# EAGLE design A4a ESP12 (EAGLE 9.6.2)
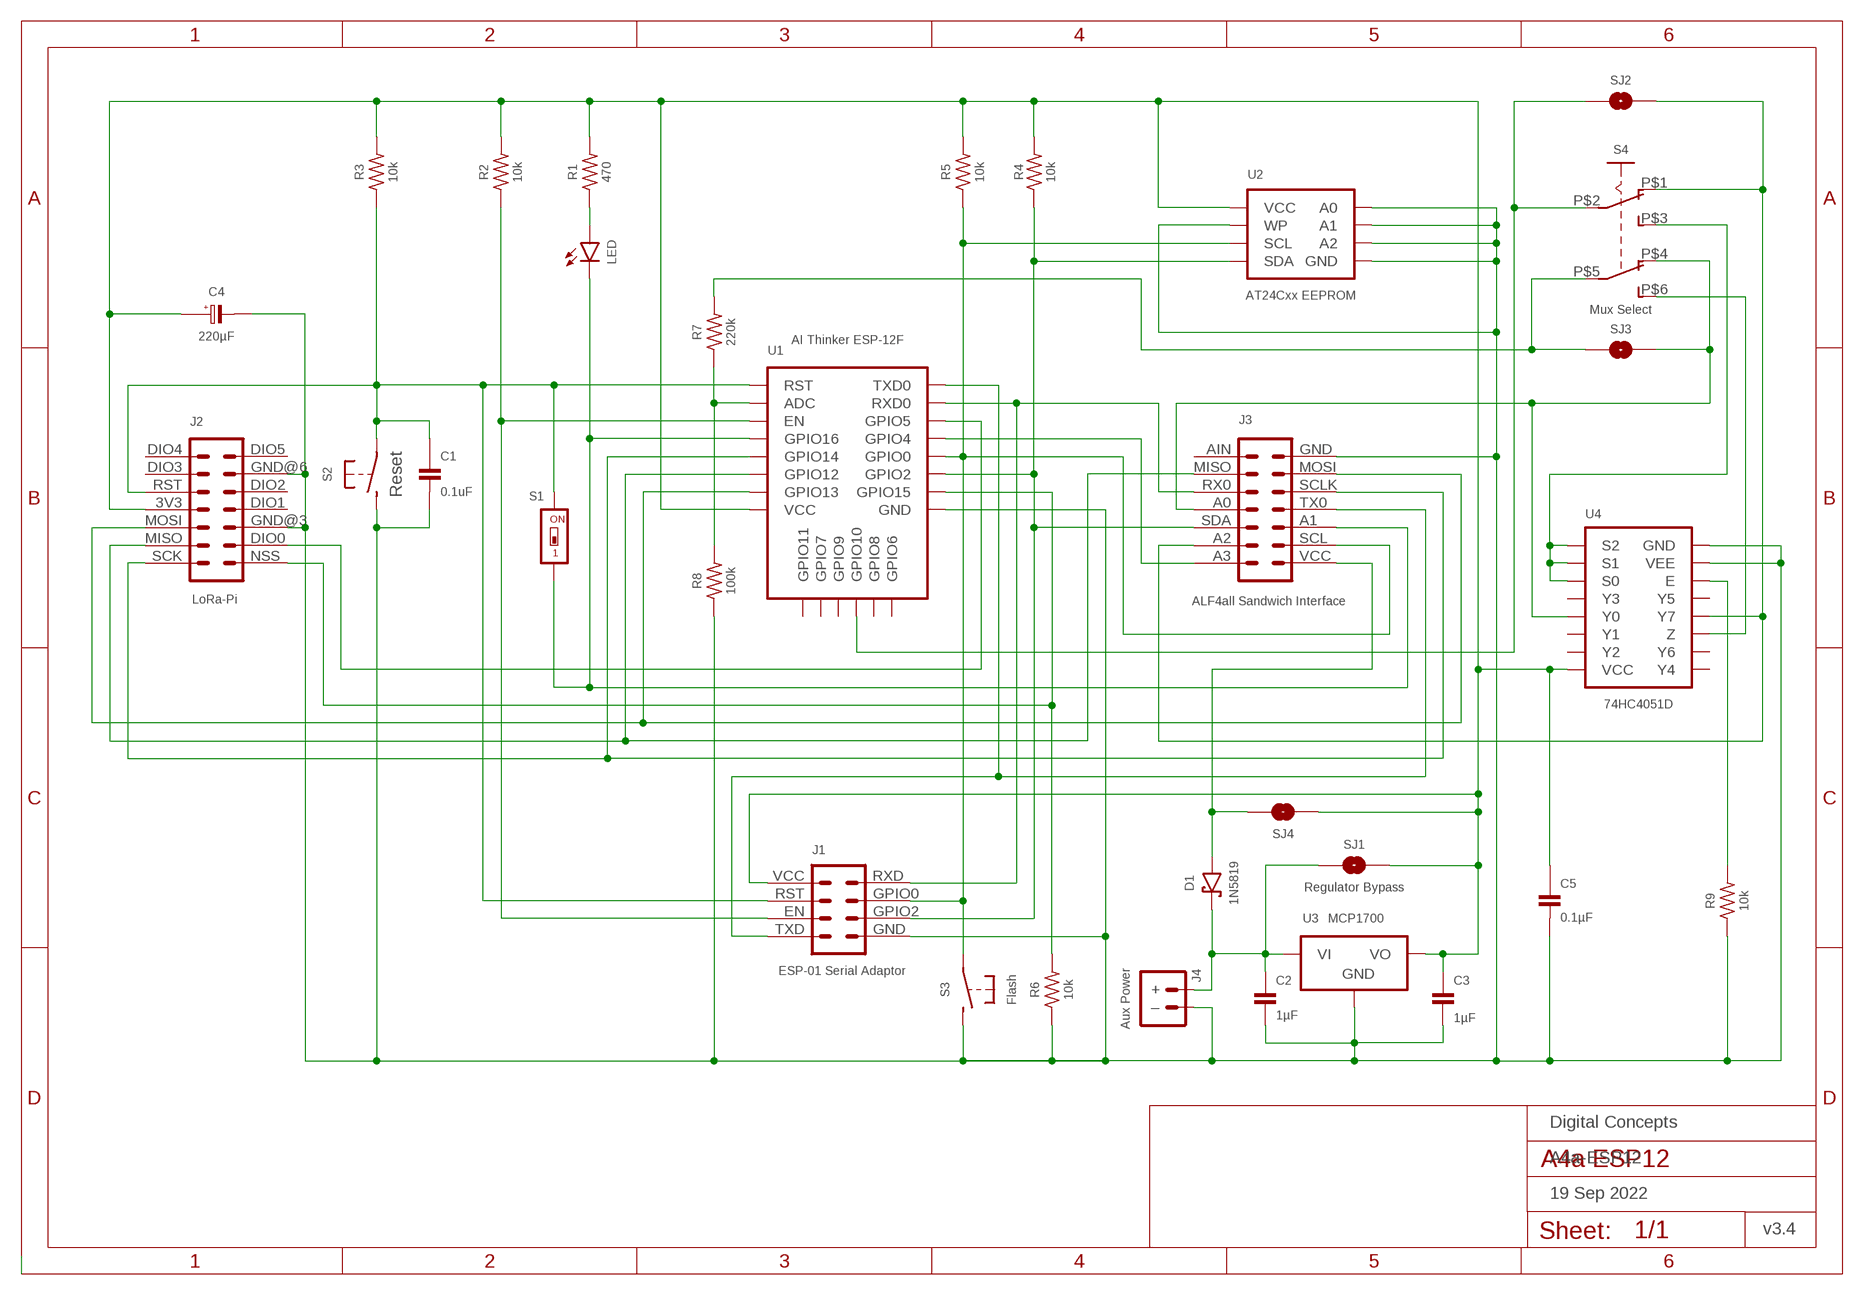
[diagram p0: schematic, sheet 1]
FRAME1 (A4L-LOC): DATE: 19 Sep 2022; OWNER: Digital Concepts; TITLE: A4a-ESP12; VERSION: v3.4

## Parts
C1  0.1uF  CAPACITOR-0805  [C0805]
C2  1µF  CAPACITOR  [C0805@1]
C3  1µF  CAPACITOR  [C0805@1]
C4  220µF  CAPACITOR-TANTALUM-3528  [C3528-21]
C5  0.1µF  CAPACITOR-0805  [C0805]
D1  1N5819  DIODE-SCHOTTKY-1N5819  [SOD-123]
J1  ESP-01 Serial Adaptor  ESP-01-SERIAL-ADAPTOR  [CONN_2X4-ESP-01-SERIAL]
J2  LoRa-Pi  RFM95W-PI-HEADER  [RFM95W-PI]
J3  ALF4all Sandwich Interface  HEADER-2X7-ALF4ALL-PROCESSOR-B  [CONN_2X7-ALF4ALL-PROCESSOR-B]
J4  Aux Power  JST-PH2.0-2-MALE-HORIZONTALJST-PTH-2  [JST-PH2.0-2-HORIZONTAL]
LED  LEDCHIP-LED0805  [CHIP-LED0805]
R1  470  RESISTORR0805  [R0805]
R2  10k  RESISTORR0805  [R0805]
R3  10k  RESISTORR0805  [R0805]
R4  10k  RESISTORR0805  [R0805]
R5  10k  RESISTORR0805  [R0805]
R6  10k  RESISTORR0805  [R0805]
R7  220k  RESISTORR0805  [R0805]
R8  100k  RESISTORR0805  [R0805]
R9  10k  RESISTORR0805  [R0805]
S1  Wake  SWITCH-DIP-SWS001  [SMD-001]
S2  Reset  SWITCH-MOMENTARY-2-PIN  [SWITCH-2-PAD]
S3  Flash  SWITCH-MOMENTARY-2-PIN  [SWITCH-2-PAD]
S4  Mux Select  SWITCH-SLIDE-DPDT  [SWITCH-DPDT-SMD]
SJ1  Regulator Bypass  SJ  [SJ]
SJ2  SJ  [SJ]
SJ3  SJ  [SJ]
SJ4  SJ  [SJ]
U1  AI Thinker ESP-12F  ESP-12E/F  [ESP-12E/F]
U2  AT24Cxx EEPROM  AT24CXX-EEPROM  [SOP-8]
U3  MCP1700  [SOT-23-3]
U4  74HC4051D  [SOP16]

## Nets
GND: C1.2 C2.2 C3.2 C4.2(-) C5.2 J1.GND J2.GND@3 J2.GND@6 J3.GND J4.-(–) R6.1 R8.1 R9.1 S2.P$2(S) S3.P$2(S) U1.GND U2.P$1(A0) U2.P$2(A1) U2.P$3(A2) U2.P$4(GND) U2.P$7(WP) U3.1(GND) U4.7(VEE) U4.8(GND)
N$1: S4.P$2(P1) SJ2.1 U1.GPIO10
N$2: J2.NSS R6.2 U1.GPIO15
N$3: J2.SCK J3.SCLK U1.GPIO14
N$4: C1.1 J1.RST J2.RST R3.1 S1.2 S2.P$1(P) U1.RST
N$5: J2.MISO J3.MISO U1.GPIO12
N$6: J2.MOSI J3.MOSI U1.GPIO13
N$7: R7.1 R8.2 U1.ADC
N$8: J1.EN R2.1 U1.EN
N$9: D1.A J3.VCC SJ4.1
N$10: J1.TXD J3.TX0 U1.TXD0
N$11: J1.GPIO2 J3.SDA R4.1 U1.GPIO2 U2.P$5(SDA)
N$12: J3.A3 U1.GPIO4
N$13: J1.GPIO0 J3.SCL R5.1 S3.P$1(P) U1.GPIO0 U2.P$6(SCL)
N$14: LED.A R1.1
N$15: J3.A1 LED.C S1.1 U1.GPIO16
N$16: J1.RXD J3.RX0 U1.RXD0
N$17: R9.2 U4.6(E)
N$19: J2.DIO0 U1.GPIO5
N$20: J3.A2 S4.P$1(O1) SJ2.2 U4.4(Y7)
N$21: J3.A0 S4.P$4(O2) SJ3.2 U4.13(Y0)
N$22: S4.P$6(S2) U4.3(Z)
N$23: S4.P$3(S1) U4.9(S2) U4.10(S1) U4.11(S0)
N$25: R7.2 S4.P$5(P2) SJ3.1
N$26: C2.1 D1.C J4.+ SJ1.1 U3.3(VI)
VCC: C3.1 C4.1(+) C5.1 J1.VCC J2.3V3 R1.2 R2.2 R3.2 R4.2 R5.2 SJ1.2 SJ4.2 U1.VCC U2.P$8(VCC) U3.2(VO) U4.16(VCC)
Unconnected: J2.DIO1 J2.DIO2 J2.DIO3 J2.DIO4 J2.DIO5 J3.AIN U1.CS0(GPIO11) U1.GPIO9 U1.MISO(GPIO7) U1.MOSI(GPIO8) U1.SCLK(GPIO6) U4.1(Y4) U4.2(Y6) U4.5(Y5) U4.12(Y3) U4.14(Y1) U4.15(Y2)

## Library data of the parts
C1 C5 = digitalconcepts:CAPACITOR-0805: 0805 Capacitor
C2 C3 = digitalconcepts:CAPACITOR: 0805 Capacitor
C4 = digitalconcepts:CAPACITOR-TANTALUM-3528: Capacitor Polarised EIA 3528-21 (KEMET B)
D1 = digitalconcepts:DIODE-SCHOTTKY-1N5819: 1N5819 Schottky Diode SOD-123
J1 = digitalconcepts:ESP-01-SERIAL-ADAPTOR: ESP-01 Serial Adpator
J2 = digitalconcepts:RFM95W-PI-HEADER: RFM95W LoRa Wireless Transceiver Raspberry Pi Daughter Board
J3 = digitalconcepts:HEADER-2X7-ALF4ALL-PROCESSOR-B: ALF4all 'Sandwich' Processor (Bottom) 2x7 Pin Header Header soldered to underside of PCB
J4 = digitalconcepts:JST-PH2.0-2-MALE-HORIZONTAL: PH2.0 2P Right Angle PCB Connector; PROD_ID: CONN-09863; SKU: PRT-09914
LED = digitalconcepts:LED: LED
R1-R9 = digitalconcepts:RESISTOR: Resistor; SPICEPREFIX: R
S1 = digitalconcepts:SWITCH-DIP-SWS001: SMD Dip Switch 1 pol.
S2 S3 = digitalconcepts:SWITCH-MOMENTARY-2-PIN: 2 Pin Momentary Switch
S4 = digitalconcepts:SWITCH-SLIDE-DPDT: Switch SMD DPDT
SJ1-SJ4 = digitalconcepts:SJ: Solder Jumper
U1 = digitalconcepts:ESP-12E/F: AI Thinker ESP-12E/F MCU
U2 = digitalconcepts:AT24CXX-EEPROM: AT24Cxx EEPROM SOP-8
U3 = digitalconcepts:MCP1700: MCP1700 Low Quiescent Current LDO Voltage Regulator
U4 = digitalconcepts:74HC4051D: 74HC4051 8-Port Multiplexer SOP-16

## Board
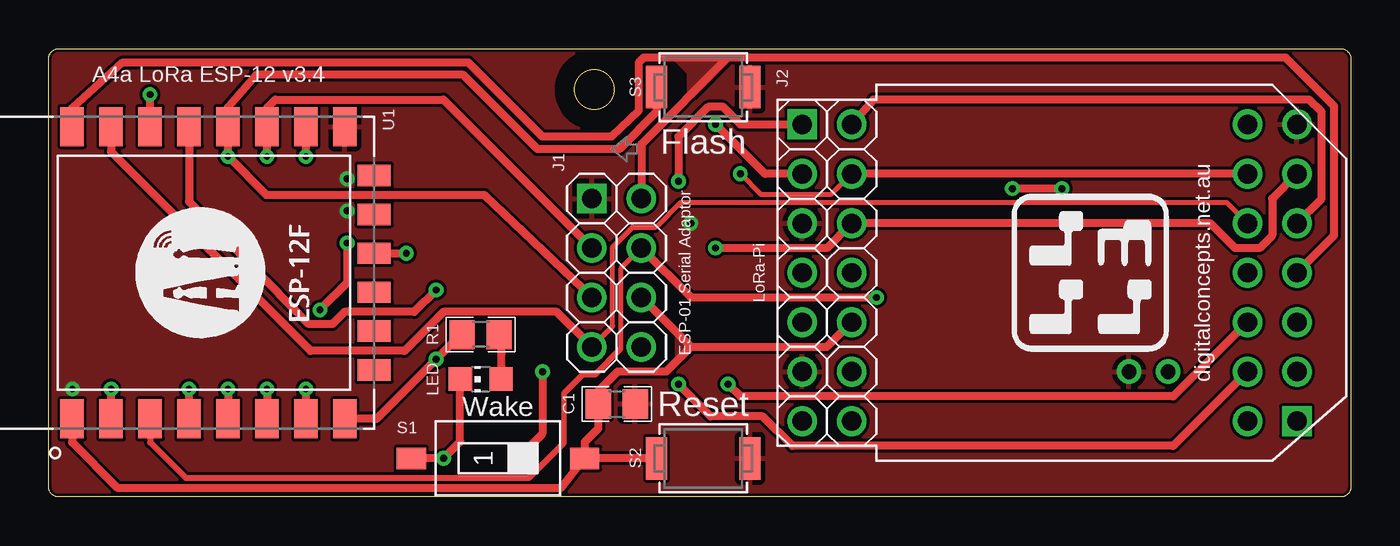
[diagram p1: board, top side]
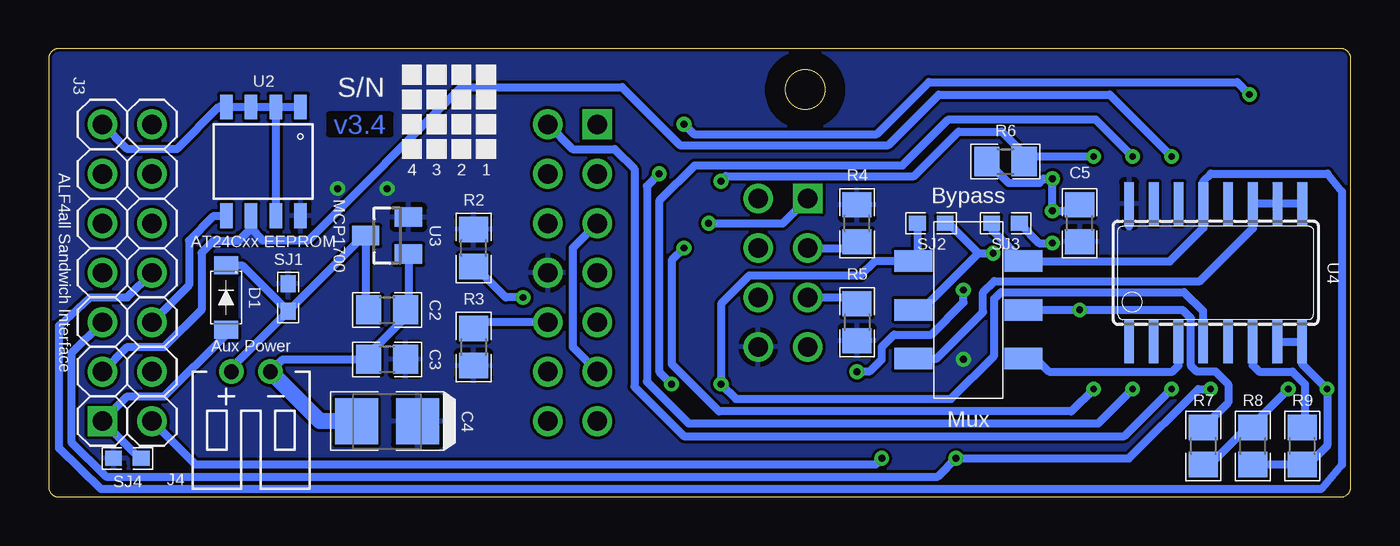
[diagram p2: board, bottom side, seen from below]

Size 66.85 x 23 mm. Coordinates in mm from the lower left corner, seen from the top.
Outline: 88 segments
Outline: circle at 28.02,20.9 radius 1.02
Copper layers (1*16): Top 0.035mm / dielectric 1.5mm / Bottom 0.035mm
Design rules "default *": minimum track width 6mil, minimum drill 0.35mm, track to track 6mil, track to pad 6mil, pad to pad 6mil, via to via 6mil, smd to smd 6mil, copper to edge 6mil, drill to drill 6mil, minimum pad ring 10mil, minimum via ring 8mil, stop-mask expansion 4mil, vias tented up to drill 0mil, thermal gap 10mil

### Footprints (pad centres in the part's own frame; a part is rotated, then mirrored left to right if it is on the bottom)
C0805 = smd 1.3 x 1.5: 1 -0.95,0; 2 0.95,0
C0805@1 = smd 1.3 x 1.5: 1 -0.95,0; 2 0.95,0
C3528-21 = smd 2.21 x 2.35: 1 -1.565,0; 2 1.565,0
SOD-123 = smd 0.91 x 1.22: A -1.65,0; C 1.65,0
CONN_2X4-ESP-01-SERIAL = drill 1 pad 1.524: EN 2.54,2.54; GPIO0 5.08,0; GPIO2 2.54,0; RST 5.08,2.54; RXD 7.62,0; TXD 0,2.54; VCC 7.62,2.54 | drill 1 pad 1.524 square: GND 0,0
RFM95W-PI = drill 1 pad 1.524: 3V3 7.62,2.54; DIO0 2.54,0; DIO1 7.62,0; DIO2 10.16,0; DIO3 12.7,2.54; DIO4 15.24,2.54; DIO5 15.24,0; GND@3 5.08,0; GND@6 12.7,0; MISO 2.54,2.54; MOSI 5.08,2.54; RST 10.16,2.54; SCK 0,2.54 | drill 1 pad 1.524 square: NSS 0,0
CONN_2X7-ALF4ALL-PROCESSOR-B = drill 1 pad 1.524: A0 7.62,2.54; A1 5.08,0; A2 2.54,2.54; A3 0,2.54; AIN 15.24,2.54; GND 15.24,0; MISO 12.7,2.54; MOSI 12.7,0; RX0 10.16,2.54; SCL 2.54,0; SCLK 10.16,0; SDA 5.08,2.54; TX0 7.62,0 | drill 1 pad 1.524 square: VCC 0,0
JST-PH2.0-2-HORIZONTAL = drill 0.75: + 1,0; - -1,0
CHIP-LED0805 = smd 1.2 x 1.2: A 0,-1.05; C 0,1.05
R0805 = smd 1.3 x 1.5: 1 -0.95,0; 2 0.95,0
SMD-001 = smd 1.1 x 1.5: 1 0,-4.45; 2 0,4.45
SWITCH-2-PAD = smd 1.067 x 2.184: P$1 -2.4,0; P$2 2.4,0
SWITCH-DPDT-SMD = smd 1.95 x 1.1: P$1 -2.825,2.5; P$2 -2.825,0; P$3 -2.825,-2.5; P$4 2.825,2.5; P$5 2.825,0; P$6 2.825,-2.5
SJ = smd 0.864 x 0.762: 1 -0.711,0; 2 0.711,0
ESP-12E/F = smd 2 x 1.2: ADC -7.5,5; EN -7.5,3; GND 7.5,-7; GPIO0 7.5,-1; GPIO2 7.5,-3; GPIO4 7.5,1; GPIO5 7.5,3; GPIO12 -7.5,-3; GPIO13 -7.5,-5; GPIO14 -7.5,-1; GPIO15 7.5,-5; GPIO16 -7.5,1; RST -7.5,7; RXD0 7.5,5; TXD0 7.5,7; VCC -7.5,-7 | smd 1.1 x 1.7: CS0 -5,-8.5; GPIO9 -1,-8.5; GPIO10 1,-8.5; MISO -3,-8.5; MOSI 3,-8.5; SCLK 5,-8.5
SOP-8 = smd 0.635 x 1.27: P$1 -1.905,-2.794; P$2 -0.635,-2.794; P$3 0.635,-2.794; P$4 1.905,-2.794; P$5 1.905,2.794; P$6 0.635,2.794; P$7 -0.635,2.794; P$8 -1.905,2.794
SOT-23-3 = smd 1 x 1.4: 1 -0.95,-1.1; 2 0.95,-1.1; 3 0,1.1
SOP16 = smd 0.5 x 2.2: 1 -4.445,-3.55; 2 -3.185,-3.55; 3 -1.915,-3.55; 4 -0.645,-3.55; 5 0.635,-3.55; 6 1.895,-3.55; 7 3.165,-3.55; 8 4.435,-3.55; 9 4.445,3.55; 10 3.175,3.55; 11 1.905,3.55; 12 0.635,3.55; 13 -0.635,3.55; 14 -1.905,3.55; 15 -3.175,3.55; 16 -4.445,3.55

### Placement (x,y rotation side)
C1  29.16,4.77 0 top
C2  49.48,9.6 0 bottom
C3  49.48,7.06 180 bottom
C4  49.48,3.88 180 bottom
C5  13.92,14.04 90 bottom
D1  57.73,10.23 90 bottom
J1  27.89,15.31 270 top
J2  38.68,19.12 270 top
J3  64.08,3.88 90 top
J4  56.46,6.42 180 bottom
LED  22.17,6.04 90 top
R1  22.17,8.33 180 top
R2  45.03,12.77 90 bottom
R3  45.03,7.69 270 bottom
R4  25.35,14.04 90 bottom
R5  25.35,8.96 270 bottom
R6  17.73,17.22 0 bottom
R7  7.57,2.61 90 bottom
R8  5.03,2.61 90 bottom
R9  2.49,2.61 90 bottom
S1  23.06,1.98 270 top
S2  33.6,1.98 0 top
S3  33.6,21.03 0 top
S4  19.63,9.6 0 bottom
SJ1  54.56,10.23 90 bottom
SJ2  21.54,14.04 180 bottom
SJ3  17.73,14.04 180 bottom
SJ4  62.81,1.98 180 bottom
U1  8.2,11.5 90 top
U2  55.83,17.22 180 bottom
U3  49.48,13.41 90 bottom
U4  6.93,11.5 0 bottom

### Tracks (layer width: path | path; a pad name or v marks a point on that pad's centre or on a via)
$X1
  cutout Top: 28.02,22.93 arc180 28.02,18.87 arc180
$X2
  cutout Bottom: 28.02,22.93 arc180 28.02,18.87 arc180
GND  (via drill 0.35)
  Bottom 0.406: U2.P$2 U2.P$3 U2.P$4 58.12,20.01 60.27,17.85 62.81,17.85 J3.GND | U2.P$2 U2.P$1 | U2.P$2 U2.P$7 | J4.- 54.83,7.06 C3.2 50.43,7.32 48.53,9.22 C2.2 48.38,9.6 U3.1 | U4.7 U4.8 2.5,6.81 v1.22,5.53 1.22,2.61 2.17,1.66 R9.1 R8.1 | J2.GND@3 39.95,12.77 39.95,7.69 J2.GND@6 | v32.97,14.04 29.16,14.04 J1.GND | R6.1 17.79,16.32 17.58,16.11 15.98,16.11 15.77,16.33 v15.32,16.33 v15.32,14.68 14.23,14.68 C5.2
  Bottom 0.813: J4.- 52.92,3.88 C4.2
  pour Top (rank 3): -1.32,24.2 67.89,24.2 67.89,-1.2 -1.32,-1.2
N$1  (via drill 0.35)
  Top 0.406: U1.GPIO10 v18.36,12.5
  Bottom 0.406: S4.P$2 22.03,9.6 19.13,12.5 | 19.13,12.5 v18.36,12.5 | 19.13,12.5 20.67,14.04 SJ2.1
N$2  (via drill 0.35)
  Top 0.406: v32.33,16.2 32.33,18.49 33.86,20.01 34.62,20.01 35.51,19.12 J2.NSS | U1.GPIO15 v13.2,17.47
  Bottom 0.406: v32.33,16.2 32.08,16.45 22.43,16.45 20.14,18.74 17.92,18.74 16.78,17.6 R6.2 16.53,17.47 v13.2,17.47
N$3  (via drill 0.35)
  Top 0.406: J3.SCLK 65.35,15.31 65.35,19.76 64.72,20.39 42.34,20.39 J2.SCK | v9.2,5.53 U1.GPIO14
  Bottom 0.406: J2.SCK 39.95,17.85 37.8,17.85 36.78,16.84 36.78,5.66 34.24,3.12 11.62,3.12 v9.2,5.53
N$4
  Top 0.406: U1.RST 1.2,2.8 3.55,0.45 26.29,0.45 S1.2 | 32.97,7.69 39.95,7.69 J2.RST | 32.97,7.69 31.7,6.42 29.21,6.42 28.21,5.42 C1.1 28.21,3.5 27.51,2.8 S1.2 | J1.RST 32.97,7.69 | S2.P$1 S1.2
  Bottom 0.406: J2.RST 44.87,8.96 R3.1
  pour Top: 32.97,7.69 32.33,8.33 32.33,7.06
N$5  (via drill 0.35)
  Top 0.254: v35.51,16.58 36.58,15.51 40.16,15.51 J2.MISO
  Top 0.406: J3.MISO J2.MISO | v11.2,5.53 U1.GPIO12
  Bottom 0.406: v35.51,16.58 36.14,15.95 36.14,5.91 33.99,3.75 12.98,3.75 v11.2,5.53
N$6  (via drill 0.35)
  Top 0.406: J3.MOSI 62.81,15.31 62.81,13.41 62.18,12.77 60.91,12.77 59.64,14.04 J2.MOSI 39.95,12.77 v34.24,12.77 | v13.2,5.53 U1.GPIO13
  Bottom 0.406: v34.24,12.77 34.87,12.14 34.87,6.83 32.44,4.39 14.35,4.39 v13.2,5.53
N$7  (via drill 0.35)
  Top 0.406: U1.ADC v3.2,5.53
  Bottom 0.406: R7.1 7.21,1.66 5.31,3.56 R8.2 5.03,3.71 v3.2,5.53
N$8  (via drill 0.35)
  Top 0.254: J1.EN 29.36,11.7 29.36,7.59
  Top 0.279: 29.36,7.59 28.04,6.27 27.41,6.27 26.45,5.32 26.45,2.78 24.64,0.96
  Top 0.305: 24.64,0.96 7.05,0.96 5.21,2.8 U1.EN
  Top 0.406: J1.EN 32.97,10.23 v42.49,10.23
  Bottom 0.406: v42.49,10.23 43.38,10.23 44.97,11.82 R2.1
N$9
  Bottom 0.406: D1.A 57.73,8.33 60.91,5.15 62.81,5.15 J3.VCC 62.18,1.98 SJ4.1
N$10
  Top 0.406: J3.TX0 65.99,13.41 65.99,20.06 63.5,22.55 34.87,22.55 | U1.TXD0 1.2,19.95 3.81,22.3 21.54,22.3 25.35,18.49 28.91,18.49 30.3,19.82 30.3,22.3 30.56,22.55 34.87,22.55 | 34.87,22.55 30.43,18.11 J1.TXD
  pour Top: 34.87,22.55 32.97,20.65 32.97,21.79 32.21,22.55
N$11  (via drill 0.35)
  Top 0.406: J3.SDA 57.73,5.15 35.51,5.15 v34.87,5.79 | J1.GPIO2 20.27,20.39 11.63,20.39 11.2,19.96 U1.GPIO2 v11.2,17.47
  Bottom 0.406: v34.87,5.79 35.51,6.42 35.51,15.18 33.68,17.01 23.01,17.01 20.65,19.38 13.11,19.38 v11.2,17.47 | J3.SDA 59.64,10.87 59.64,13.15 58.37,14.42 U2.P$5 | R4.1 25.67,12.77 J1.GPIO2
N$12  (via drill 0.35)
  Top 0.406: U1.GPIO4 7.2,15.15 13.35,8.86 14.55,8.86 15.19,9.49 18.77,9.49 v19.89,10.61 | v25.35,6.42 25.35,3.25 v24.08,1.98
  Bottom 0.406: J3.A3 59.33,1.67 24.38,1.67 v24.08,1.98 | v25.35,6.42 24.71,6.42 24.08,7.06 24.08,7.69 23.44,8.33 21.54,8.33 19.89,9.98 v19.89,10.61
N$13  (via drill 0.35)
  Top 0.406: J1.GPIO0 22.38,15.49 11.19,15.49 v9.2,17.47 U1.GPIO0 9.2,20.02 10.65,21.66 21.29,21.66 25.1,17.85 29.3,17.85 31.2,19.76 S3.P$1
  Bottom 0.406: J3.SCL 62.81,7.69 60.91,7.69 59,9.6 59,12.52 58.37,13.15 57.1,13.15 56.46,13.79 | U2.P$6 56.46,13.79 | v9.2,17.47 12.38,20.65 21.16,20.65 23.75,18.05 34.44,18.05 37.41,21.03 45.67,21.03 53.54,13.15 55.83,13.15 56.46,13.79 | J1.GPIO0 25.67,10.23 R5.1
  pour Bottom: 56.46,13.79 57.1,13.15 55.83,13.15
N$14
  Top 0.406: R1.1 23.22,8.23 LED.A
N$15  (via drill 0.35)
  Top 0.406: U1.GPIO16 v7.2,5.53 | S1.1 v20.27,1.98 21.12,2.83 LED.C
  Bottom 0.406: v7.2,5.53 7.84,5.53 11.4,1.98 v20.27,1.98 21.21,1.04 63.91,1.04 65.68,2.81 65.68,7.36 J3.A1
N$16
  Top 0.254: J3.RX0 60.48,15.11 32.45,15.11 31.18,13.84 29.97,13.84 28.96,12.82 28.96,8.76 J1.RXD
  Top 0.406: J1.RXD 26.09,9.49 20.27,9.49 18.26,7.49 13.44,7.49 3.2,17.72 U1.RXD0
N$17
  Bottom 0.406: R9.2 2.36,3.69 2.36,5.79 3,6.42 4.71,6.42 5.04,6.75 U4.6
N$19  (via drill 0.35)
  Top 0.406: J2.DIO0 36.78,16.58 v34.24,19.12 | U1.GPIO5 v5.2,20.65
  Bottom 0.406: v5.2,20.65 5.84,21.28 21.67,21.28 24.33,18.61 33.73,18.61 v34.24,19.12
N$20  (via drill 0.35)
  Top 0.406: v32.33,5.79 33.99,4.14 36.65,4.14 38.18,2.61 57.73,2.61 J3.A2
  Bottom 0.406: U4.4 7.58,9.53 8.56,10.51 17.96,10.51 18.3,10.17 18.3,7.25 20.52,5.02 31.57,5.02 v32.33,5.79 32.33,9.91 30.89,11.35 25.19,11.35 24.44,12.1 S4.P$1 22.25,12.31 SJ2.2
N$21
  Bottom 0.406: J3.A0 62.81,10.23 64.72,10.23 66.32,8.78 66.32,2.48 64.16,0.4 1.52,0.4 0.46,1.64 0.46,15.66 1.21,16.59 7.19,16.59 7.57,16.21 U4.13 7.57,13.81 9.29,12.09 14.82,12.09 14.83,12.1 S4.P$4 18.44,13.73 SJ3.2
N$22
  Bottom 0.406: S4.P$6 16.17,7.1 15.5,6.42 9.16,6.42 8.85,6.73 U4.3
N$23
  Bottom 0.406: U4.9 U4.10 U4.11 5.03,13.78 7.74,11.07 18.31,11.07 18.88,10.5 18.88,9.48 21.27,7.1 S4.P$3
N$25  (via drill 0.35)
  Top 0.406: v15.32,13.03 15.32,10.99 v13.92,9.6
  Bottom 0.406: R7.2 6.3,4.83 6.3,5.79 6.93,6.42 7.9,6.42 8.2,6.72 8.2,9.16 8.64,9.6 v13.92,9.6 S4.P$5 | SJ3.1 16,13.03 v15.32,13.03
N$26
  Bottom 0.406: C2.1 50.58,9.75 U3.3 50.67,13.41 SJ1.1 | J4.+ 57.46,6.62 SJ1.1 | D1.C 56.92,11.88 SJ1.1
VCC  (via drill 0.35)
  Top 0.406: U1.VCC 16.83,4 v19.89,7.06 21.16,8.33 R1.2 | v52.02,15.82 v49.48,15.82
  Bottom 0.406: U4.16 11.38,13.88
  pour Bottom (rank 3): -0.69,23.57 67.26,23.57 67.26,-0.56 -0.69,-0.56

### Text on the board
Bottom: v3.4
tPlace: A4a LoRa ESP-12 v3.4 | digitalconcepts.net.au
bPlace: S/N | 1 | 2 | 3 | 4
bNames: Bypass | Mux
